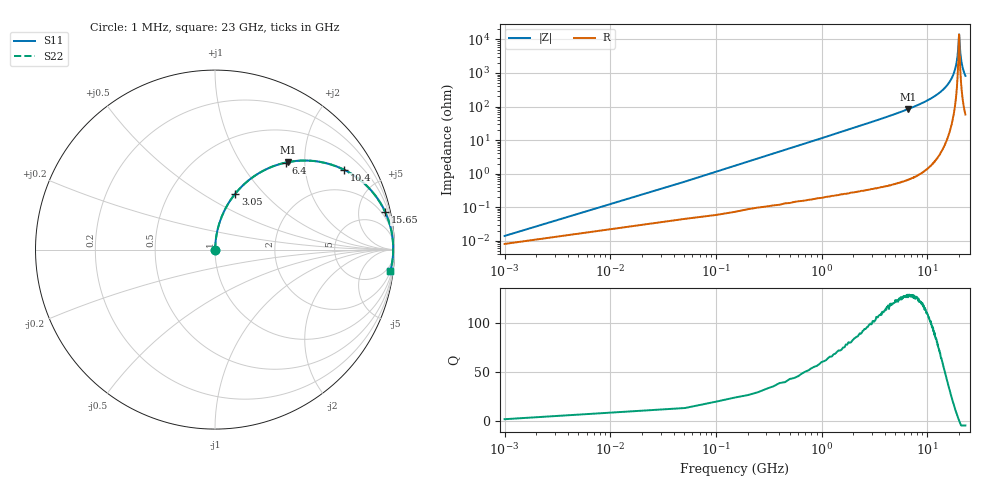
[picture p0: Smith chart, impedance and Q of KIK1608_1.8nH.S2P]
!version-2
!date-01.2022
!Series
# MHz S RI R 50
!Freq ReS11 ImS11 ReS21 ImS21 ReS12 ImS12 ReS22 ImS22
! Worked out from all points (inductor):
!   461 points, 1 MHz to 23 GHz, reference 50 ohm
!   read as one part in series: L = 1.8 nH near 101 MHz
!   highest Q = 128 at 6.55 GHz (marker M1), where L = 2.02 nH
!   self-resonance near 20 GHz
!   S11 on the Smith chart (normalised r, x): 1 MHz: 1.00, +0.00; 3.05 GHz: 1.01, +0.71; 6.4 GHz: 1.01, +1.61; 10.4 GHz: 1.03, +3.22; 15.65 GHz: 1.24, +9.05; 23 GHz: 2, -16
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1  6.01e-05 0.000113  0.9999 -0.000113  0.9999 -0.000113  6.01e-05 0.000113
151  0.00103 0.017  0.999 -0.017  0.999 -0.017  0.00103 0.017
301  0.00219 0.0339  0.9978 -0.0339  0.9978 -0.0339  0.00219 0.0339
501  0.00453 0.0564  0.9955 -0.0564  0.9955 -0.0564  0.00453 0.0564
851  0.0109 0.0952  0.9891 -0.0952  0.9891 -0.0952  0.0109 0.0952
1400  0.0268 0.1546  0.9732 -0.1546  0.9732 -0.1546  0.0268 0.1546
3050  0.1133 0.3121  0.8867 -0.3121  0.8867 -0.3121  0.1133 0.3121
3850  0.172 0.3729  0.828 -0.3729  0.828 -0.3729  0.172 0.3729
6400  0.3947 0.4849  0.6053 -0.4849  0.6053 -0.4849  0.3947 0.4849
6550  0.4083 0.4876  0.5917 -0.4876  0.5917 -0.4876  0.4083 0.4876
7700  0.5106 0.4959  0.4894 -0.4959  0.4894 -0.4959  0.5106 0.4959
10400  0.7196 0.4445  0.2804 -0.4445  0.2804 -0.4445  0.7196 0.4445
11550  0.7901 0.4018  0.2099 -0.4018  0.2099 -0.4018  0.7901 0.4018
15350  0.9415 0.2231  0.0585 -0.2231  0.0585 -0.2231  0.9415 0.2231
15650  0.9486 0.2082  0.0514 -0.2082  0.0514 -0.2082  0.9486 0.2082
17850  0.9835 0.1004  0.0165 -0.1004  0.0165 -0.1004  0.9835 0.1004
19200  0.9918 0.0376  0.00816 -0.0376  0.00816 -0.0376  0.9918 0.0376
19550  0.9927 0.022  0.00735 -0.022  0.00735 -0.022  0.9927 0.022
20050  0.9929 -2.59e-06  0.00707 2.59e-06  0.00707 2.59e-06  0.9929 -2.59e-06
20600  0.9921 -0.0235  0.00786 0.0235  0.00786 0.0235  0.9921 -0.0235
21100  0.9905 -0.0443  0.0095 0.0443  0.0095 0.0443  0.9905 -0.0443
23000  0.9774 -0.1176  0.0226 0.1176  0.0226 0.1176  0.9774 -0.1176
